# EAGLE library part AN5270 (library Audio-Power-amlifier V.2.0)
4.3 W ´ 1(8W) Power Amplifier with Volume Control and Tone Control
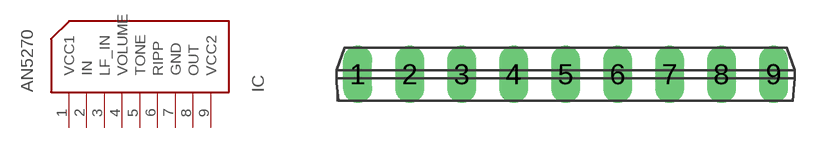
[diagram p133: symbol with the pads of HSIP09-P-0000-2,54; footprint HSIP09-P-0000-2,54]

Designator prefix IC

## AN5270  [HSIP09-P-0000-2,54]
1  VCC1  pwr
2  IN  in
3  LF_IN  in
4  VOLUME  in
5  TONE  in
6  RIPP
7  GND  pwr
8  OUT  out
9  VCC2  pwr

## Footprint HSIP09-P-0000-2,54 (pad centres in mm)
drill 0.9 long: 1 -10.16,0; 2 -7.62,0; 3 -5.08,0; 4 -2.54,0; 5 0,0; 6 2.54,0; 7 5.08,0; 8 7.62,0; 9 10.16,0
